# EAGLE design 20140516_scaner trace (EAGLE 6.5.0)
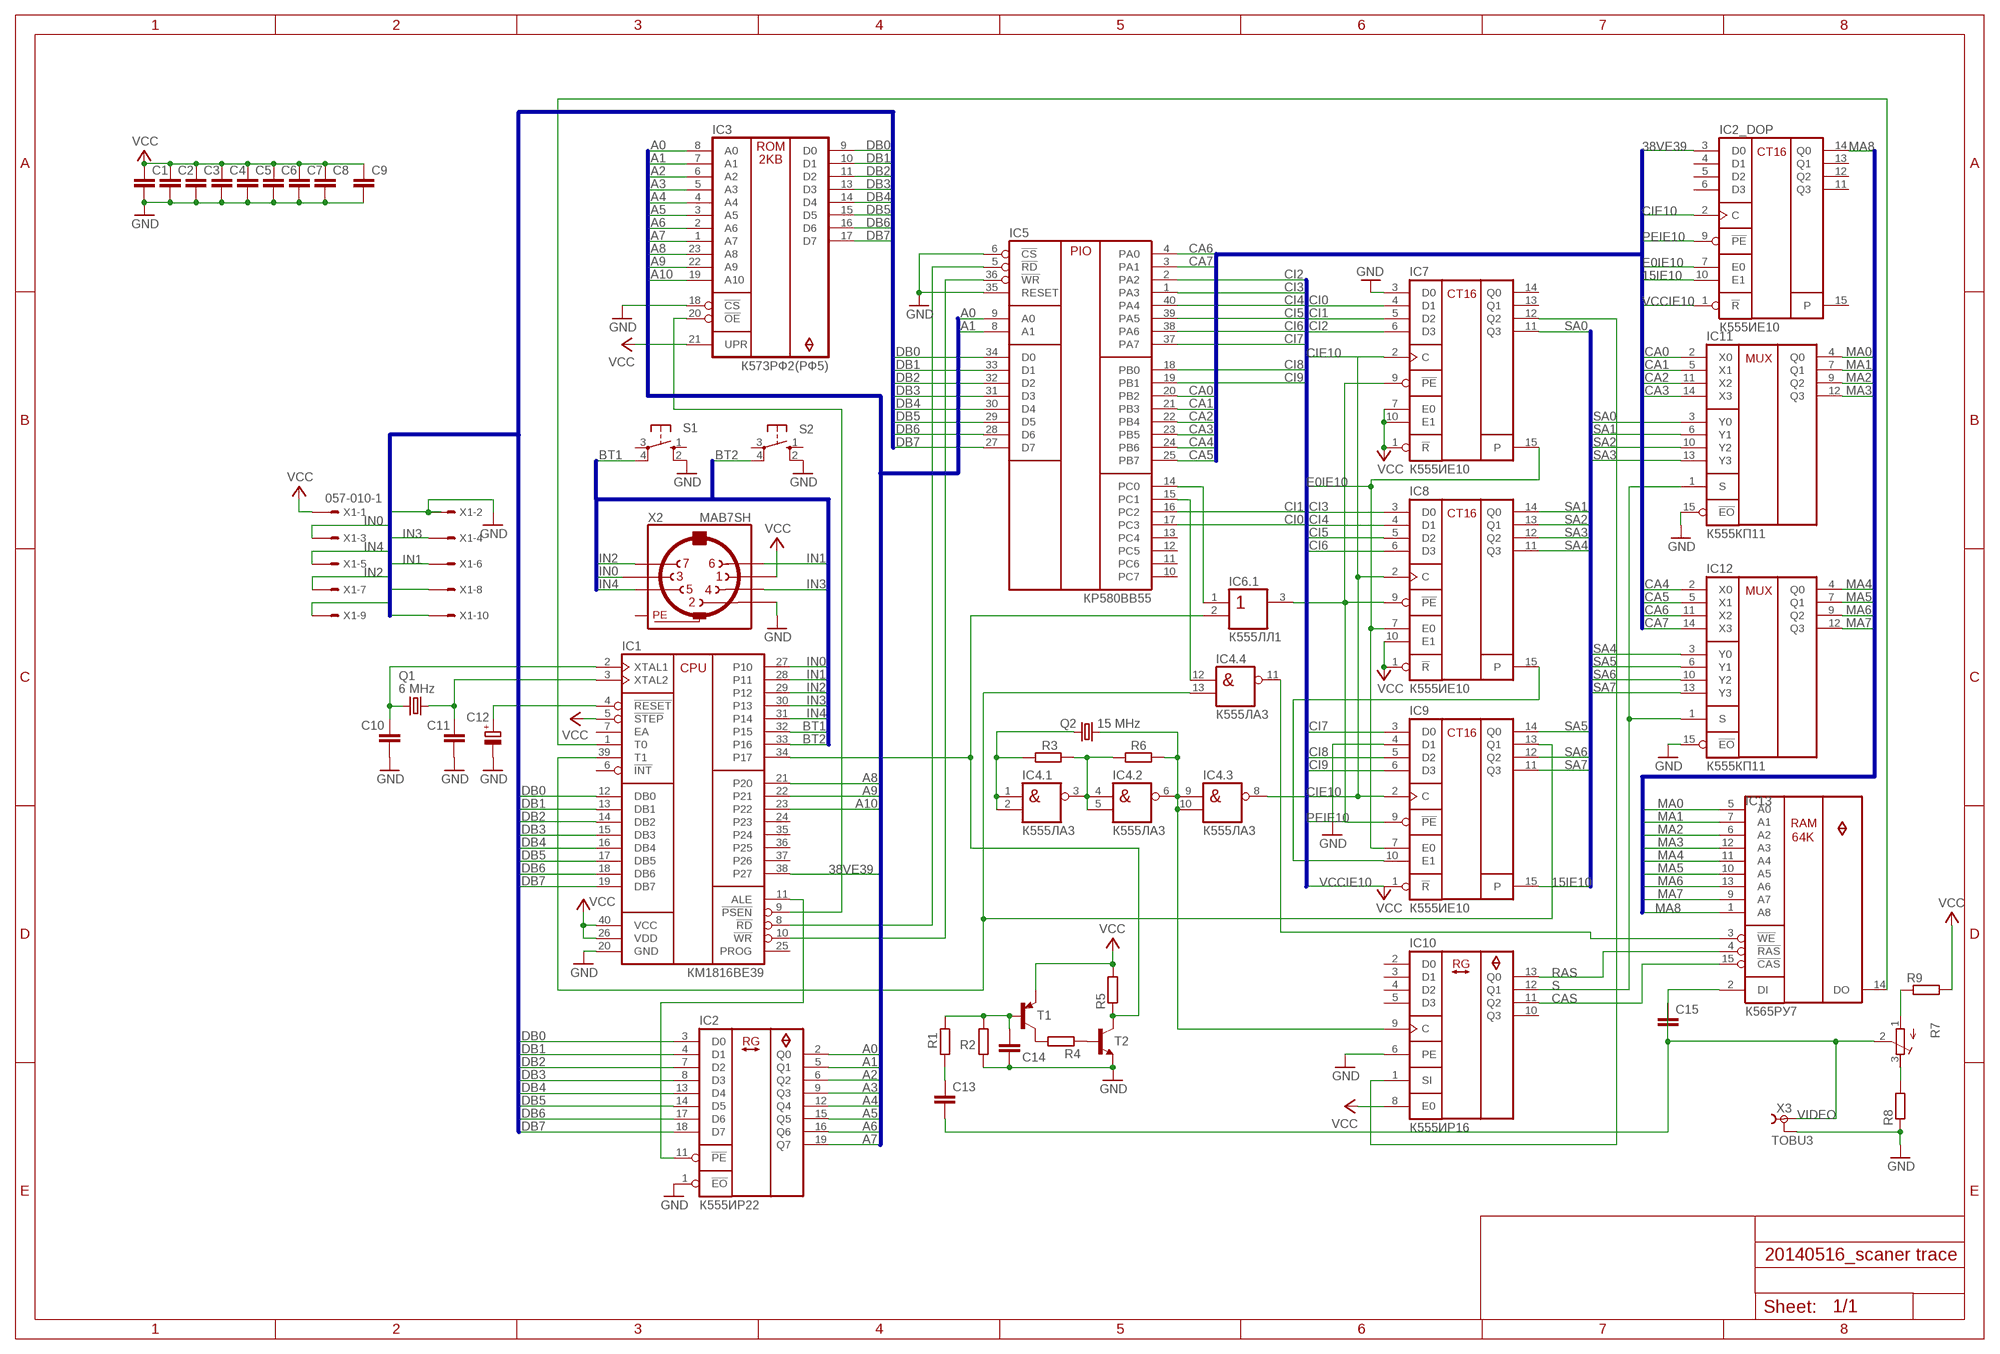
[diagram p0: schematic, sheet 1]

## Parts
C1  C-EU050-025X075  [C050-025X075]
C2  C-EU050-025X075  [C050-025X075]
C3  C-EU050-025X075  [C050-025X075]
C4  C-EU050-025X075  [C050-025X075]
C5  C-EU050-025X075  [C050-025X075]
C6  C-EU050-025X075  [C050-025X075]
C7  C-EU050-025X075  [C050-025X075]
C8  C-EU050-025X075  [C050-025X075]
C9  C-EU050-025X075  [C050-025X075]
C10  C-EU050-025X075  [C050-025X075]
C11  C-EU050-025X075  [C050-025X075]
C12  CPOL-EUE2,5-6E  [E2,5-6E]
C13  C-EU050-025X075  [C050-025X075]
C14  C-EU050-025X075  [C050-025X075]
C15  C-EU050-025X075  [C050-025X075]
IC1  КМ1816ВЕ39  [DIP40]
IC2  К555ИР22  [DIP20]
IC2_DOP  К555ИЕ10  [DIP16]
IC3  К573РФ2(РФ5)  К573РФ2  [DIP24]
IC4  К555ЛА3  [DIP14]
IC5  КР580ВВ55  [DIP40]
IC6  К555ЛЛ1  [DIP14]
IC7  К555ИЕ10  [DIP16]
IC8  К555ИЕ10  [DIP16]
IC9  К555ИЕ10  [DIP16]
IC10  К555ИР16  [DIP14]
IC11  К555КП11  [DIP16]
IC12  К555КП11  [DIP16]
IC13  К565РУ7  [DIP16]
Q1  6 MHz  CRYSTALZX_V  [HC49U_V_ZX]
Q2  15 MHz  CRYSTALZX_V  [HC49U_V_ZX]
R1  R-EU_  [0207/10_L17]
R2  R-EU_  [0207/10_L17]
R3  R-EU_  [0207/10_L17]
R4  R-EU_  [0207/10_L17]
R5  R-EU_  [0207/10_L17]
R6  R-EU_  [0207/10_L17]
R7  R-TRIMM3339P  [RTRIM3339P]
R8  R-EU_  [0207/10_L17]
R9  R-EU_  [0207/10_L17]
S1  40-XX  [B3F-40XX-LION17]
S2  40-XX  [B3F-40XX-LION17]
T1  -PNP-  [TO92-EBC-LION17]
T2  -NPN-  [KT315]
X1  057-010-1  [057-010-1]
X2  MAB7SH  [DIN7]
X3  TOBU3  [TOBU3]

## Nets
15IE10: IC2_DOP.10(E1) IC9.15(P)
38VE39: IC1.38(P27) IC2_DOP.3(D0)
A0: IC2.2(Q0) IC3.8(A0) IC5.9(A0)
A1: IC2.5(Q1) IC3.7(A1) IC5.8(A1)
A2: IC2.6(Q2) IC3.6(A2)
A3: IC2.9(Q3) IC3.5(A3)
A4: IC2.12(Q4) IC3.4(A4)
A5: IC2.15(Q5) IC3.3(A5)
A6: IC2.16(Q6) IC3.2(A6)
A7: IC2.19(Q7) IC3.1(A7)
A8: IC1.21(P20) IC3.23(A8)
A9: IC1.22(P21) IC3.22(A9)
A10: IC1.23(P22) IC3.19(A10)
BT1: IC1.32(P15) S1.4(P1)
BT2: IC1.33(P16) S2.4(P1)
CA0: IC5.20(PB2) IC11.2(X0)
CA1: IC5.21(PB3) IC11.5(X1)
CA2: IC5.22(PB4) IC11.11(X2)
CA3: IC5.23(PB5) IC11.14(X3)
CA4: IC5.24(PB6) IC12.2(X0)
CA5: IC5.25(PB7) IC12.5(X1)
CA6: IC5.4(PA0) IC12.11(X2)
CA7: IC5.3(PA1) IC12.14(X3)
CAS: IC10.11(Q2) IC13.15(!CAS)
CI0: IC5.17(PC3) IC7.4(D1)
CI1: IC5.16(PC2) IC7.5(D2)
CI2: IC5.2(PA2) IC7.6(D3)
CI3: IC5.1(PA3) IC8.3(D0)
CI4: IC5.40(PA4) IC8.4(D1)
CI5: IC5.39(PA5) IC8.5(D2)
CI6: IC5.38(PA6) IC8.6(D3)
CI7: IC5.37(PA7) IC9.3(D0)
CI8: IC5.18(PB0) IC9.5(D2)
CI9: IC5.19(PB1) IC9.6(D3)
CIE10: IC2_DOP.2(C) IC4.8(.3:OUT) IC7.2(C) IC8.2(C) IC9.2(C)
DB0: IC1.12(DB0) IC2.3(D0) IC3.9(D0) IC5.34(D0)
DB1: IC1.13(DB1) IC2.4(D1) IC3.10(D1) IC5.33(D1)
DB2: IC1.14(DB2) IC2.7(D2) IC3.11(D2) IC5.32(D2)
DB3: IC1.15(DB3) IC2.8(D3) IC3.13(D3) IC5.31(D3)
DB4: IC1.16(DB4) IC2.13(D4) IC3.14(D4) IC5.30(D4)
DB5: IC1.17(DB5) IC2.14(D5) IC3.15(D5) IC5.29(D5)
DB6: IC1.18(DB6) IC2.17(D6) IC3.16(D6) IC5.28(D6)
DB7: IC1.19(DB7) IC2.18(D7) IC3.17(D7) IC5.27(D7)
E0IE10: IC2_DOP.7(E0) IC7.15(P) IC8.7(E0) IC9.7(E0)
GND [GND]: C1.2 C2.2 C3.2 C4.2 C5.2 C6.2 C7.2 C8.2 C9.2 C10.2 C11.2 C12.- C14.2 IC1.20(GND) IC2.1(!EO) IC3.18(!CS) IC5.6(!CS) IC5.35(RESET) IC7.3(D0) IC9.4(D1) IC10.6(PE) IC11.15(!EO) IC12.15(!EO) R2.1 R8.1 S1.2(S1) S2.2(S1) T2.E X1.2 X2.2 X3.2 X3.2@1 X3.2@2
IN0: IC1.27(P10) X1.3 X2.3
IN1: IC1.28(P11) X1.6 X2.6
IN2: IC1.29(P12) X1.7 X2.7
IN3: IC1.30(P13) X1.4 X2.4
IN4: IC1.31(P14) X1.5 X2.5
MA0: IC11.4(Q0) IC13.5(A0)
MA1: IC11.7(Q1) IC13.7(A1)
MA2: IC11.9(Q2) IC13.6(A2)
MA3: IC11.12(Q3) IC13.12(A3)
MA4: IC12.4(Q0) IC13.11(A4)
MA5: IC12.7(Q1) IC13.10(A5)
MA6: IC12.9(Q2) IC13.13(A6)
MA7: IC12.12(Q3) IC13.9(A7)
MA8: IC2_DOP.14(Q0) IC13.1(A8)
N$1: IC8.15(P) IC9.10(E1)
N$4: C13.2 C15.2
N$6: X1.9
N$11: X1.8
N$12: X1.10
N$14: IC7.12(Q2) IC10.1(SI)
N$15: IC4.1(.1:IN1) IC4.2(.1:IN2) Q2.1 R3.1
N$16: IC4.3(.1:OUT) IC4.4(.2:IN1) IC4.5(.2:IN2) R3.2 R6.1
N$17: IC4.6(.2:OUT) IC4.9(.3:IN1) IC4.10(.3:IN2) IC10.9(C) Q2.2 R6.2
N$38: IC5.14(PC0) IC6.1(.1:IN1)
N$39: IC4.12(.4:IN1) IC5.15(PC1)
N$66: IC1.1(T0) IC13.14(DO)
N$67: C13.1 R1.2
N$69: R7.3(A) R8.2
N$70: R7.1(E) R9.1
N$71: C14.1 R1.1 R2.2 T1.B
N$72: C10.1 IC1.2(XTAL1) Q1.1
N$73: IC1.39(T1) IC4.13(.4:IN2) IC9.13(Q1)
N$74: C11.1 IC1.3(XTAL2) Q1.2
N$75: C12.+ IC1.4(!RESET)
N$76: IC1.8(!RD) IC5.5(!RD)
N$77: IC1.9(!PSEN) IC3.20(!OE)
N$78: IC1.10(!WR) IC5.36(!WR)
N$79: IC1.11(ALE) IC2.11(!PE)
N$85: IC1.34(P17) IC6.2(.1:IN2) R5.1 T2.C
N$86: R4.1 T2.B
N$87: R4.2 T1.C
PEIE10: IC2_DOP.9(!PE) IC6.3(.1:OUT) IC7.9(!PE) IC8.9(!PE) IC9.9(!PE)
RAS: IC10.13(Q0) IC13.4(!RAS)
S: IC10.12(Q1) IC11.1(S) IC12.1(S)
SA0: IC7.11(Q3) IC11.3(Y0)
SA1: IC8.14(Q0) IC11.6(Y1)
SA2: IC8.13(Q1) IC11.10(Y2)
SA3: IC8.12(Q2) IC11.13(Y3)
SA4: IC8.11(Q3) IC12.3(Y0)
SA5: IC9.14(Q0) IC12.6(Y1)
SA6: IC9.12(Q2) IC12.10(Y2)
SA7: IC9.11(Q3) IC12.13(Y3)
VCC [+5V]: C1.1 C2.1 C3.1 C4.1 C5.1 C6.1 C7.1 C8.1 C9.1 IC1.5(!STEP) IC1.26(VDD) IC1.40(VCC) IC3.21(UPR) IC7.1(!R) IC7.7(E0) IC7.10(E1) IC8.1(!R) IC8.10(E1) IC10.8(E0) R5.2 R9.2 T1.E X1.1 X2.1
VCCIE10: IC2_DOP.1(!R) IC9.1(!R) ; supply symbol labelled VCC
VIDEO: C15.1 IC13.2(DI) R7.2(S) X3.1
WE: IC4.11(.4:OUT) IC13.3(!WE)
Unconnected: IC1.6(!INT) IC1.7(EA) IC1.24(P23) IC1.25(PROG) IC1.35(P24) IC1.36(P25) IC1.37(P26) IC2_DOP.4(D1) IC2_DOP.5(D2) IC2_DOP.6(D3) IC2_DOP.11(Q3) IC2_DOP.12(Q2) IC2_DOP.13(Q1) IC2_DOP.15(P) IC5.10(PC7) IC5.11(PC6) IC5.12(PC5) IC5.13(PC4) IC6.4(.2:IN1) IC6.5(.2:IN2) IC6.6(.2:OUT) IC6.8(.3:OUT) IC6.9(.3:IN1) IC6.10(.3:IN2) IC6.11(.4:OUT) IC6.12(.4:IN1) IC6.13(.4:IN2) IC7.13(Q1) IC7.14(Q0) IC10.2(D0) IC10.3(D1) IC10.4(D2) IC10.5(D3) IC10.10(Q3) S1.1(S) S1.3(P) S2.1(S) S2.3(P) X2.PE X2.PE1(PE) X2.PE@1(PE) X2.PE@(PE)

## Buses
DB[0..7]
MA[0..7]
CA[0..7]
SA[0..7]
CI[0..9]
A[0..10]
IN[0..4],BT[1..2]

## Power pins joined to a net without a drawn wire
GND: IC2.10(GND) IC2_DOP.8(GND) IC3.12(GND) IC4.7(GND) IC5.7(GND) IC6.7(GND) IC7.8(GND) IC8.8(GND) IC9.8(GND) IC10.7(GND) IC11.8(GND) IC12.8(GND)
VCC: IC2.20(VCC) IC2_DOP.16(VCC) IC3.24(VCC) IC4.14(VCC) IC5.26(VCC) IC6.14(VCC) IC7.16(VCC) IC8.16(VCC) IC9.16(VCC) IC10.14(VCC) IC11.16(VCC) IC12.16(VCC)

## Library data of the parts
C1-C11 C13-C15 = rcl:C-EU: CAPACITOR, European symbol
C12 = rcl:CPOL-EU: POLARIZED CAPACITOR, European symbol
IC1 = lion17:КМ1816ВЕ39
IC2 = lion17:К555ИР22
IC2_DOP = _lion17:К555ИЕ10
IC3 = lion17:К573РФ2
IC4 = lion17:К555ЛА3
IC5 = lion17:КР580ВВ55
IC6 = lion17:К555ЛЛ1
IC7-IC9 = lion17:К555ИЕ10
IC10 = lion17:К555ИР16
IC11 IC12 = lion17:К555КП11
IC13 = _lion17:К565РУ7
Q1 Q2 = crystal:CRYSTAL: CRYSTAL
R1-R6 R8 R9 = rcl:R-EU_: RESISTOR, European symbol
R7 = resistor:R-TRIMM: Trimm resistor
S1 S2 = switch-omron:40-XX: OMRON SWITCH
T1 = transistor-neu-to92:*-PNP-: PNP Transistror
T2 = transistor-neu-to92:*-NPN-: NPN Transistror
X1 = con-panduit:057-010-: CONNECTOR 10-pin series 057 contact pc board low profile headers; OC_FARNELL: unknown; OC_NEWARK: unknown
X2 = con-hirschmann:MAB7SH: Female CONNECTOR 7 pins with shield, horizontal (DIN 45329)
X3 = con-hirschmann:TOBU3: Female Cinch CONNECTOR ( RCA Jack ); MF: FARNELL; MPN: TOBU 3; OC_FARNELL: 592791; OC_NEWARK: 06WX5914

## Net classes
0 default: clearance 0.205 mm
1 GND: width 0.203 mm, clearance 0.205 mm to class 0, clearance 0.205 mm
2 +5V: width 0.203 mm, clearance 0.205 mm to class 0, clearance 0.205 mm to class 1, clearance 0.205 mm

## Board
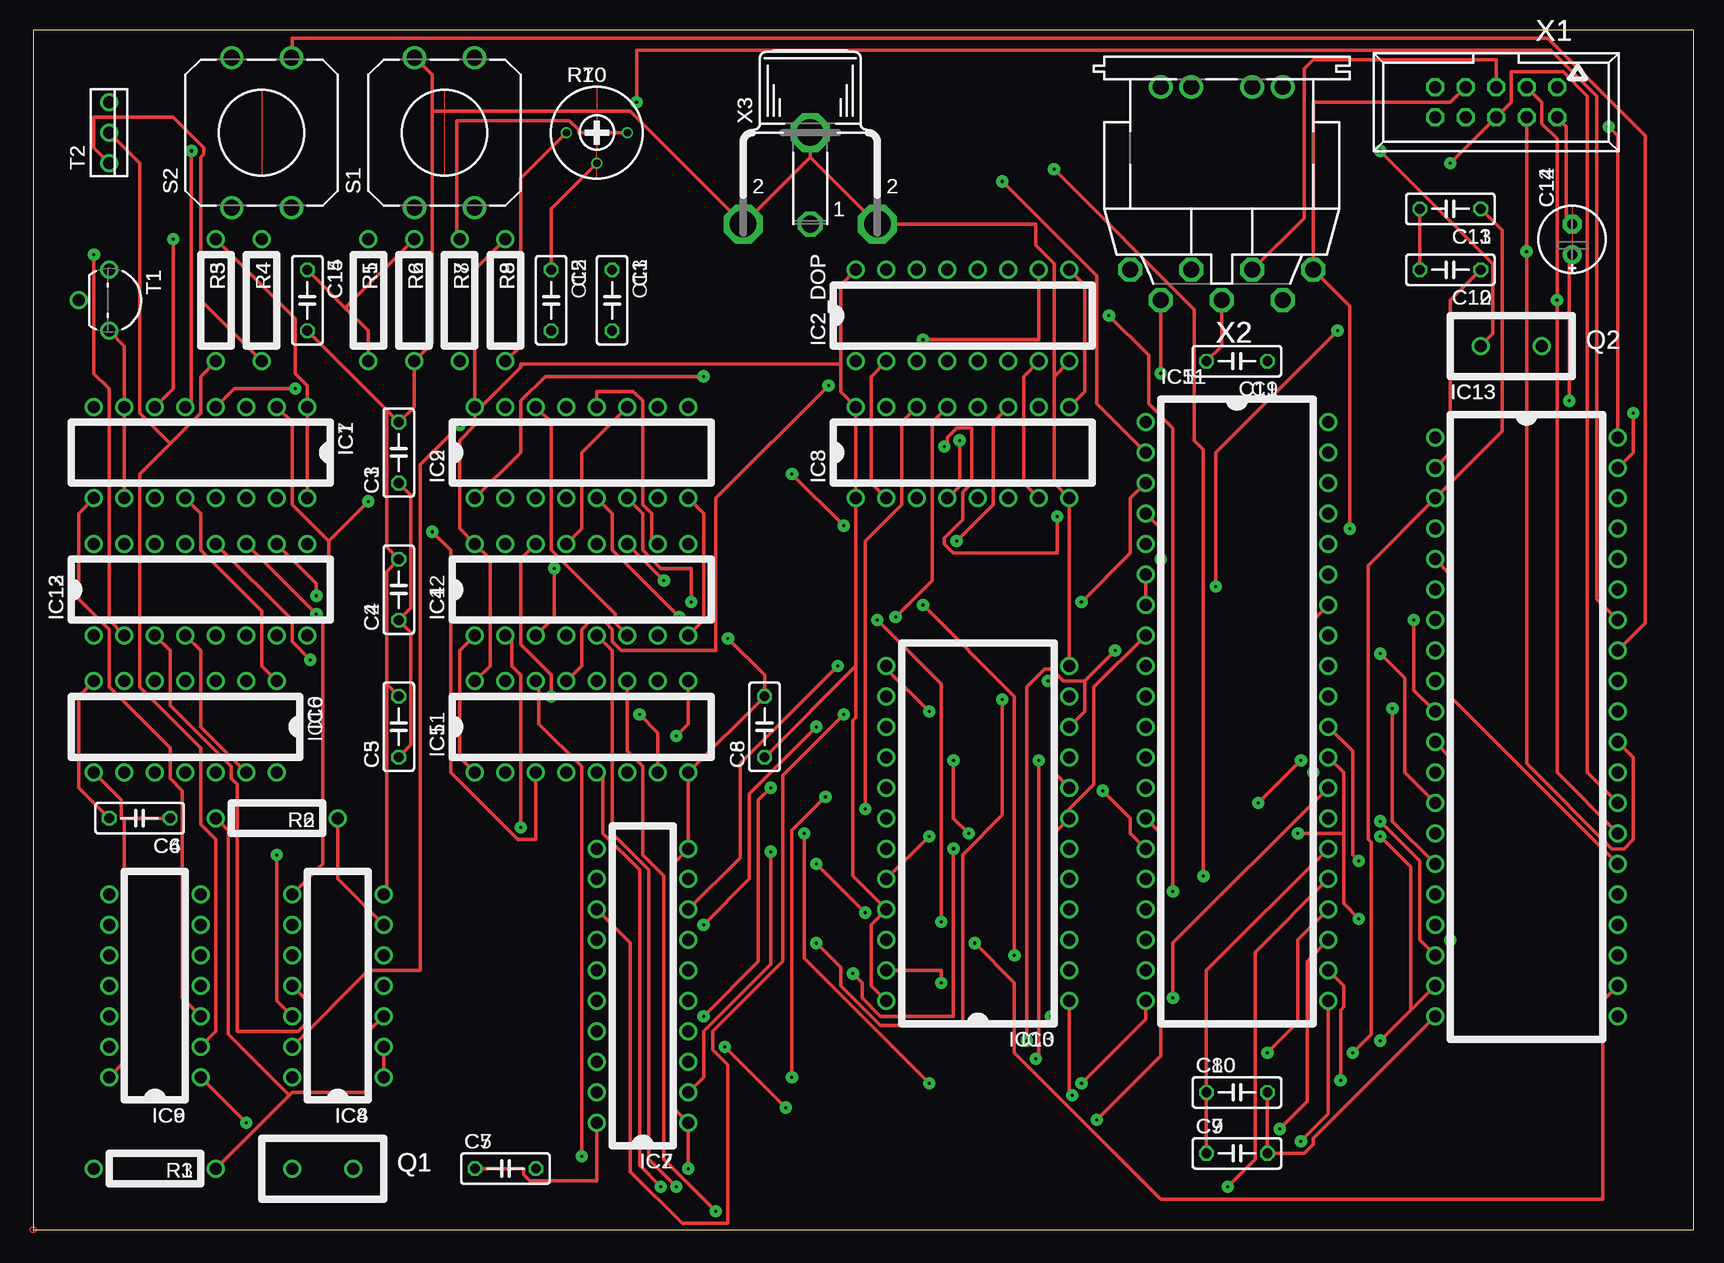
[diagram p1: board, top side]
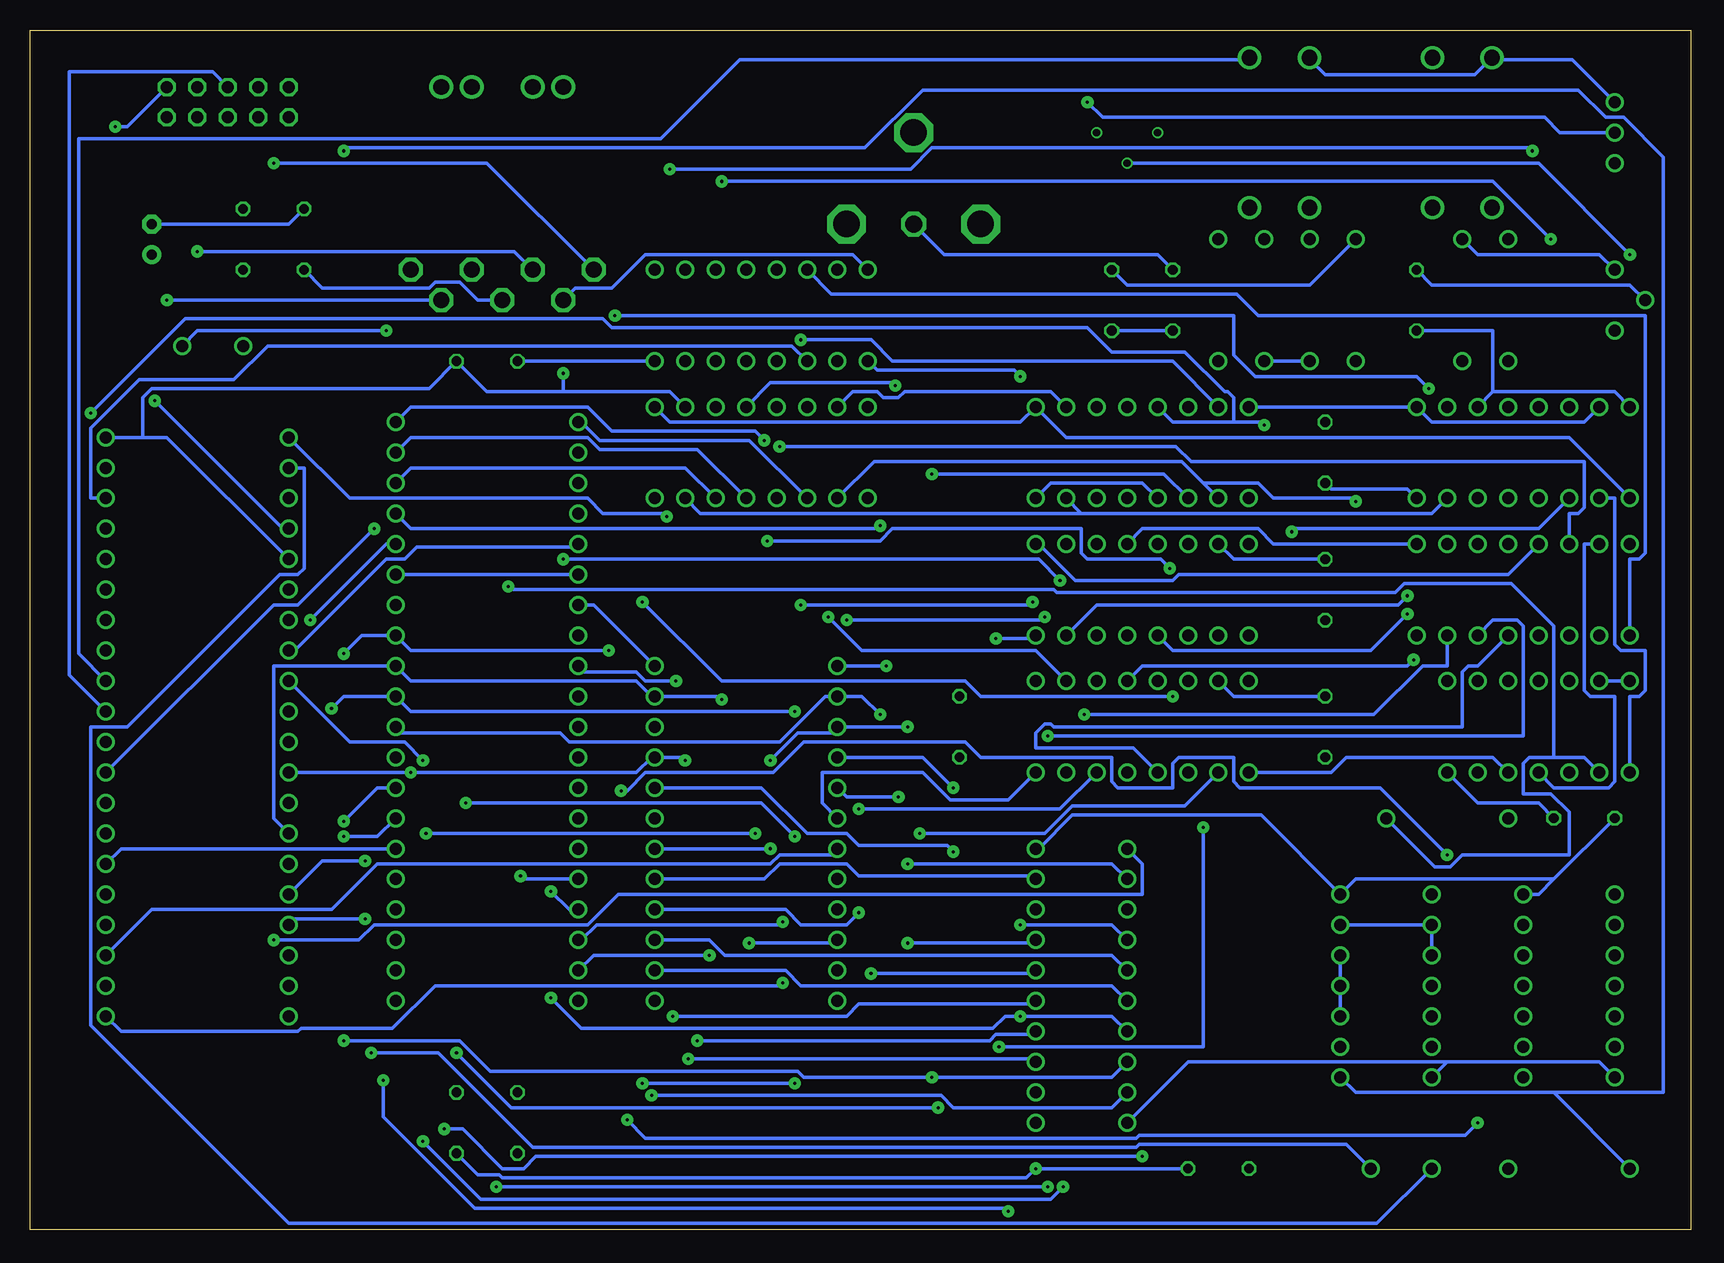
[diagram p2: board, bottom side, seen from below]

Size 138.41 x 100 mm. Coordinates in mm from the lower left corner, seen from the top.
Outline: 0,0 138.41,0 138.41,100 0,100 0,0
Copper layers (1*16): Top 0.035mm / dielectric 1.5mm / Bottom 0.035mm
Design rules "20140516_scaner trace": minimum track width 12mil, minimum drill 10mil, track to track 0.205mm, track to pad 0.205mm, pad to pad 0.205mm, via to via 0.205mm, smd to smd 8mil, copper to edge 10mil, drill to drill 20mil, minimum pad ring 5mil, minimum via ring 15mil, stop-mask expansion 4mil, vias tented up to drill 0mil, thermal gap 10mil

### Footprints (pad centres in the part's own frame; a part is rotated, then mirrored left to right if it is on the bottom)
C050-025X075 = drill 0.813 octagon: 1 -2.54,0; 2 2.54,0
E2,5-6E = drill 0.813 pad 1.575: + -1.27,0 | drill 0.813 pad 1.575 octagon: - 1.27,0
DIP40 = drill 1 pad 1.422: 1 -7.62,2.54; 2 -7.62,0; 3 -7.62,-2.54; 4 -7.62,-5.08; 5 -7.62,-7.62; 6 -7.62,-10.16; 7 -7.62,-12.7; 8 -7.62,-15.24; 9 -7.62,-17.78; 10 -7.62,-20.32; 11 -7.62,-22.86; 12 -7.62,-25.4; 13 -7.62,-27.94; 14 -7.62,-30.48; 15 -7.62,-33.02; 16 -7.62,-35.56; 17 -7.62,-38.1; 18 -7.62,-40.64; 19 -7.62,-43.18; 20 -7.62,-45.72; 21 7.62,-45.72; 22 7.62,-43.18; 24 7.62,-38.1; 25 7.62,-35.56; 26 7.62,-33.02; 27 7.62,-30.48; 28 7.62,-27.94; 29 7.62,-25.4; 30 7.62,-22.86; 31 7.62,-20.32; 32 7.62,-17.78; 33 7.62,-15.24; 34 7.62,-12.7; 35 7.62,-10.16; 36 7.62,-7.62; 37 7.62,-5.08; 38 7.62,-2.54; 39 7.62,0; 40 7.62,2.54 | drill 1: 23 7.62,-40.64
DIP20 = drill 1 pad 1.422: 1 -3.81,1.27; 2 -3.81,-1.27; 3 -3.81,-3.81; 4 -3.81,-6.35; 5 -3.81,-8.89; 6 -3.81,-11.43; 7 -3.81,-13.97; 8 -3.81,-16.51; 9 -3.81,-19.05; 10 -3.81,-21.59; 11 3.81,-21.59; 12 3.81,-19.05; 13 3.81,-16.51; 14 3.81,-13.97; 15 3.81,-11.43; 16 3.81,-8.89; 17 3.81,-6.35; 18 3.81,-3.81; 19 3.81,-1.27; 20 3.81,1.27
DIP16 = drill 1 pad 1.422: 1 -3.81,1.27; 2 -3.81,-1.27; 3 -3.81,-3.81; 4 -3.81,-6.35; 5 -3.81,-8.89; 6 -3.81,-11.43; 7 -3.81,-13.97; 8 -3.81,-16.51; 9 3.81,-16.51; 10 3.81,-13.97; 11 3.81,-11.43; 12 3.81,-8.89; 13 3.81,-6.35; 14 3.81,-3.81; 15 3.81,-1.27; 16 3.81,1.27
DIP24 = drill 1 pad 1.422: 1 -7.62,1.27; 2 -7.62,-1.27; 3 -7.62,-3.81; 4 -7.62,-6.35; 5 -7.62,-8.89; 6 -7.62,-11.43; 7 -7.62,-13.97; 8 -7.62,-16.51; 9 -7.62,-19.05; 10 -7.62,-21.59; 11 -7.62,-24.13; 12 -7.62,-26.67; 13 7.62,-26.67; 14 7.62,-24.13; 15 7.62,-21.59; 16 7.62,-19.05; 17 7.62,-16.51; 18 7.62,-13.97; 19 7.62,-11.43; 20 7.62,-8.89; 21 7.62,-6.35; 22 7.62,-3.81; 23 7.62,-1.27; 24 7.62,1.27
DIP14 = drill 1 pad 1.422: 1 -3.81,1.27; 2 -3.81,-1.27; 3 -3.81,-3.81; 4 -3.81,-6.35; 5 -3.81,-8.89; 6 -3.81,-11.43; 7 -3.81,-13.97; 8 3.81,-13.97; 9 3.81,-11.43; 10 3.81,-8.89; 11 3.81,-6.35; 12 3.81,-3.81; 13 3.81,-1.27; 14 3.81,1.27
HC49U_V_ZX = drill 1 pad 1.422: 1 -2.54,0; 2 2.54,0
0207/10_L17 = drill 1 pad 1.422: 1 -5.08,0; 2 5.08,0
RTRIM3339P = drill 0.61: 1 -2.54,0; 2 0,-2.54; 3 2.54,0
B3F-40XX-LION17 = drill 1.3: 1 -6.248,2.489; 2 6.248,2.489; 3 -6.248,-2.489; 4 6.248,-2.489
TO92-EBC-LION17 = drill 1 pad 1.422: B 0,-2.54; C -2.54,0; E 2.54,0
KT315 = drill 1 pad 1.422: B -2.54,0; C 0,0; E 2.54,0
057-010-1 = drill 1 octagon: 1 -5.08,-1.27; 2 -5.08,1.27; 3 -2.54,-1.27; 4 -2.54,1.27; 5 0,-1.27; 6 0,1.27; 7 2.54,-1.27; 8 2.54,1.27; 9 5.08,-1.27; 10 5.08,1.27
DIN7 = drill 1.321 octagon: 1 5.08,12.7; 2 0,12.7; 3 -5.08,12.7; 4 2.54,10.16; 5 -2.54,10.16; 6 7.62,10.16; 7 -7.62,10.16 | drill 1.321: PE -2.54,-5.08; PE1 -5.08,-5.08; PE@ 2.54,-5.08; PE@1 5.08,-5.08
TOBU3 = drill 1.397 octagon: 1 0,-2.54 | drill 2.21 octagon: 2 5.588,-2.54; 2@1 -5.588,-2.54; 2@2 0,5.08

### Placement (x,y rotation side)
C1  30.48,64.77 90 top
C2  30.48,53.34 90 top
C3  30.48,41.91 90 top
C4  8.89,34.29 180 top
C5  39.37,5.08 0 top
C6  60.96,41.91 90 top
C7  100.33,6.35 0 top
C8  100.33,11.43 0 top
C9  100.33,72.39 180 top
C10  118.11,80.01 180 top
C11  118.11,85.09 180 top
C12  128.27,82.55 90 top
C13  48.26,77.47 270 top
C14  22.86,77.47 270 top
C15  43.18,77.47 270 top
DRILEGEND  [DRILEGEND]  not placed on the board
IC1  124.46,63.5 0 top
IC2  50.8,10.16 180 top
IC2_DOP  69.85,76.2 90 top
IC3  78.74,20.32 180 top
IC4  25.4,13.97 180 top
IC5  100.33,64.77 0 top
IC6  10.16,13.97 180 top
IC7  21.59,64.77 270 top
IC8  69.85,64.77 90 top
IC9  38.1,64.77 90 top
IC10  19.05,41.91 270 top
IC11  38.1,41.91 90 top
IC12  38.1,53.34 90 top
IC13  6.35,53.34 90 top
Q1  24.13,5.08 0 top
Q2  123.19,73.66 0 top
R1  27.94,77.47 90 top
R2  31.75,77.47 90 top
R3  10.16,5.08 0 top
R4  19.05,77.47 90 top
R5  15.24,77.47 90 top
R6  20.32,34.29 0 top
R7  46.99,91.44 0 top
R8  35.56,77.47 90 top
R9  39.37,77.47 90 top
S1  34.29,91.44 90 top
S2  19.05,91.44 90 top
T1  6.35,77.47 270 top
T2  6.35,91.44 90 top
X1  121.92,93.98 180 top
X2  99.06,90.17 180 top
X3  64.77,86.36 0 top

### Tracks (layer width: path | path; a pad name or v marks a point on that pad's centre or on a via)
15IE10  (via drill 0.25)
  Top 0.305: v74.17,74.17 83.82,74.17 IC2_DOP.10
  Bottom 0.305: IC9.15 43.18,72.39 66.55,72.39 68.33,74.17 v74.17,74.17
38VE39
  Bottom 0.305: IC2_DOP.3 74.93,73.66 118.62,73.66 121.41,70.87 129.29,70.87 133.35,66.8 133.35,60.96 IC1.38
A0  (via drill 0.25)
  Top 0.305: IC2.2 55.88,12.7 55.88,16.51 61.47,22.1 v61.47,31.5 | v84.58,45.72 85.09,45.21 85.09,38.1 IC3.8
  Bottom 0.305: v61.47,31.5 61.98,32 69.34,32 70.36,33.02 73.66,33.02 77.47,36.83 IC3.8 | IC5.9 92.2,46.48 87.88,46.48 87.12,45.72 v84.58,45.72
A1  (via drill 0.25)
  Top 0.305: v84.84,17.78 85.09,18.03 85.09,33.02 IC3.7 86.36,35.05 88.39,37.08 88.39,45.21 IC5.8
  Bottom 0.305: IC2.5 54.86,18.8 69.34,18.8 70.36,17.78 v84.84,17.78
A2  (via drill 0.25)
  Top 0.305: v68.33,21.34 69.09,20.57 69.09,19.3 70.61,17.78 76.71,17.78 v76.71,31.75
  Bottom 0.305: IC2.6 54.86,21.34 v68.33,21.34 | IC3.6 v76.71,31.75
A3
  Bottom 0.305: IC2.9 54.86,29.46 69.34,29.46 70.36,30.48 75.95,30.48 77.22,29.21 IC3.5
A4  (via drill 0.25)
  Top 0.305: v69.34,26.42 v65.28,30.48
  Bottom 0.305: IC2.12 48.26,30.48 v65.28,30.48 | v69.34,26.42 70.36,25.4 74.17,25.4 75.44,26.67 IC3.4
A5
  Bottom 0.305: IC2.15 48.26,22.86 80.52,22.86 81.79,24.13 IC3.3
A6
  Bottom 0.305: IC2.16 48.26,20.32 74.17,20.32 75.44,21.59 IC3.2
A7  (via drill 0.25)
  Top 0.305: v86.61,11.18 86.36,11.43 IC3.1
  Bottom 0.305: IC2.19 48.26,10.16 61.47,10.16 62.48,11.18 v86.61,11.18
A8  (via drill 0.25)
  Top 0.305: IC3.23 75.69,21.59 v75.69,20.57
  Bottom 0.305: v75.69,20.57 75.95,20.32 104.65,20.32 108.2,16.76 115.82,16.76 116.08,16.51 130.81,16.51 IC1.21
A9  (via drill 0.25)
  Top 0.305: v78.49,23.88 81.79,20.57 81.79,14.73 93.98,2.54 130.81,2.54 130.81,19.05 IC1.22
  Bottom 0.305: IC3.22 71.37,23.88 v78.49,23.88
A10
  Bottom 0.305: IC3.19 71.63,31.24 75.95,31.24 76.71,30.48 109.47,30.48 113.28,26.67 128.27,26.67 IC1.23
BT1
  Bottom 0.305: IC1.32 134.37,48.01 134.37,90.93 85.85,90.93 79.25,97.54 36.83,97.54 S1.4
BT2
  Top 0.305: IC1.33 134.37,50.55 134.37,91.19 126.24,99.31 21.59,99.31 21.59,97.79 S2.4
CA0  (via drill 0.25)
  Top 0.305: v64.26,33.02 64.26,22.61 v74.68,12.19 | v87.38,12.19 92.71,17.53 IC5.20
  Bottom 0.305: IC11.2 42.16,35.31 51.56,35.31 53.85,33.02 v64.26,33.02 | v87.38,12.19 v74.68,12.19
CA1  (via drill 0.25)
  Top 0.305: IC11.5 47.5,37.59 47.5,33.02 50.55,29.97 50.55,5.33 v52.32,3.56 | v105.66,7.37 107.95,9.65 IC5.21
  Bottom 0.305: v52.32,3.56 53.34,2.54 100.84,2.54 v105.66,7.37
CA2  (via drill 0.25)
  Top 0.305: IC11.11 49.53,39.88 50.8,38.61 50.8,31.24 52.58,29.46 52.58,5.84 v56.9,1.52 | v108.97,12.45 108.97,18.29 109.22,18.54 109.22,20.32 IC5.22
  Bottom 0.305: v56.9,1.52 57.15,1.78 101.35,1.78 108.97,9.4 v108.97,12.45
CA3  (via drill 0.25)
  Top 0.305: IC11.14 42.16,45.47 42.16,42.16 45.72,38.61 v45.72,6.1 | v103.89,8.38 106.17,10.67 106.17,22.35 IC5.23
  Bottom 0.305: v45.72,6.1 96.27,6.1 97.28,5.08 99.06,5.08 102.36,8.38 v103.89,8.38
CA4  (via drill 0.25)
  Top 0.305: IC12.2 39.88,49.02 39.88,46.99 40.64,46.23 v40.64,33.53 | v62.74,10.16 v57.66,15.24 | v102.87,14.73 105.41,17.27 105.41,24.13 IC5.24
  Bottom 0.305: v40.64,33.53 40.64,15.24 v57.66,15.24 | v62.74,10.16 98.3,10.16 v102.87,14.73
CA5  (via drill 0.25)
  Top 0.305: IC12.5 48.26,48.26 48.26,33.02 51.31,29.97 51.31,5.84 v53.59,3.56 | v99.57,3.56 101.85,5.84 101.85,23.11 IC5.25
  Bottom 0.305: v99.57,3.56 v53.59,3.56
CA6  (via drill 0.25)
  Top 0.305: v52.58,54.1 IC12.11 | v93.98,55.88 93.98,58.42 IC5.4
  Bottom 0.305: v52.58,54.1 54.36,55.88 v93.98,55.88
CA7  (via drill 0.25)
  Top 0.305: IC12.14 40.64,55.88 40.64,48.77 43.18,46.23 v43.18,44.45 | v87.38,52.32 91.44,56.39 91.44,60.96 IC5.3
  Bottom 0.305: v43.18,44.45 59.18,44.45 60.45,45.72 80.77,45.72 v87.38,52.32
CAS
  Bottom 0.305: IC10.11 11.43,36.83 6.86,36.83 6.35,37.34 6.35,44.45 8.38,44.45 8.89,44.96 8.89,57.15 IC13.15
CI0  (via drill 0.25)
  Top 0.305: IC7.4 16.76,70.1 v21.84,70.1 | v89.66,76.2 92.96,72.9 92.96,68.83 95,66.8 v95,28.19
  Bottom 0.305: v21.84,70.1 22.86,71.12 36.32,71.12 38.1,72.9 38.1,76.2 v89.66,76.2 | v95,28.19 93.47,26.67 IC5.17
CI1  (via drill 0.25)
  Top 0.305: IC7.5 13.21,69.09 v13.21,89.92 | v85.09,88.39 96.77,76.71 96.77,65.79 97.54,65.02 v97.54,29.46
  Bottom 0.305: v13.21,89.92 13.46,90.17 63.25,90.17 65.02,88.39 v85.09,88.39 | v97.54,29.46 97.28,29.21 IC5.16
CI2  (via drill 0.25)
  Top 0.305: IC7.6 11.68,70.1 v11.68,82.55 | v80.77,87.38 88.65,79.5 88.65,68.83 IC5.2
  Bottom 0.305: v11.68,82.55 16.51,87.38 v80.77,87.38
CI3
  Bottom 0.305: IC8.3 78.49,65.79 90.93,65.79 92.46,67.31 IC5.1
CI4  (via drill 0.25)
  Top 0.305: IC8.4 77.22,61.98 v77.22,65.79
  Bottom 0.305: v77.22,65.79 77.98,66.55 89.92,66.55 91.95,68.58 106.68,68.58 IC5.40
CI5
  Bottom 0.305: IC8.5 82.8,65.02 90.93,65.02 91.95,66.04 106.68,66.04 IC5.39
CI6
  Bottom 0.305: IC8.6 83.82,63.5 106.68,63.5 IC5.38
CI7  (via drill 0.25)
  Top 0.305: v67.56,58.67 v63.25,62.99
  Bottom 0.305: IC9.3 43.94,62.99 v63.25,62.99 | v67.56,58.67 67.82,58.42 106.68,58.42 IC5.37
CI8  (via drill 0.25)
  Top 0.305: IC9.5 48.26,59.69 48.26,56.64 v53.85,51.05 | v70.36,50.8 75.69,45.47 v75.69,25.65
  Bottom 0.305: v53.85,51.05 54.1,50.8 v70.36,50.8 | v75.69,25.65 75.95,25.4 91.19,25.4 92.46,24.13 IC5.18
CI9  (via drill 0.25)
  Top 0.305: IC9.6 50.8,59.69 50.8,56.64 52.32,55.12 54.86,55.12 v54.86,52.32 | v74.17,52.07 81.79,44.45 v81.79,22.86
  Bottom 0.305: v54.86,52.32 55.12,52.07 v74.17,52.07 | v81.79,22.86 91.44,22.86 IC5.19
CIE10  (via drill 0.25)
  Top 0.305: IC4.8 24.13,30.48 24.13,50.55 24.64,51.05 24.64,57.4 | 24.64,57.4 21.59,60.45 21.59,67.31 IC7.2 | IC2_DOP.2 69.85,71.12 69.85,62.23 IC8.2 | v27.94,60.71 24.64,57.4
  Bottom 0.305: 40.64,62.23 42.42,64.01 68.07,64.01 IC8.2 | 40.64,62.23 IC9.2 | v27.94,60.71 28.19,60.96 34.8,60.96 36.07,62.23 40.64,62.23
DB0  (via drill 0.25)
  Top 0.305: v83.57,14.22 83.82,14.48 v83.82,39.12 | IC5.34 106.68,50.8 v106.68,38.1
  Bottom 0.305: IC2.3 54.86,14.22 v83.57,14.22 | v83.82,39.12 84.07,39.37 IC3.9 86.61,39.37 87.88,38.1 v106.68,38.1 IC1.12
DB1  (via drill 0.25)
  Top 0.305: IC1.13 114.3,38.1 114.3,45.97 v112.27,48.01 | v82.8,15.75 82.8,45.21 84.33,46.74 85.09,46.74 85.09,46.48 85.85,45.72 87.63,45.72 | 87.63,45.72 87.63,43.18 IC3.10 | 87.63,45.72 v90.17,48.26
  Bottom 0.305: v112.27,48.01 110.74,49.53 IC5.33 106.68,48.26 v90.17,48.26 | IC2.4 54.86,16.26 57.91,16.26 58.42,15.75 v82.8,15.75
DB2  (via drill 0.25)
  Top 0.305: v65.28,23.88 67.31,21.84 67.31,20.32 70.61,17.02 77.47,17.02 77.47,31.24 80.77,34.54 v80.77,44.2
  Bottom 0.305: IC2.7 54.86,23.88 v65.28,23.88 | v80.77,44.2 81.03,44.45 IC3.11 86.61,44.45 87.88,45.72 106.68,45.72 IC5.32 118.11,46.99 118.11,34.29 IC1.14
DB3  (via drill 0.25)
  Top 0.305: IC1.15 113.28,34.04 v113.28,43.43 | IC2.8 58.93,30.99 58.93,38.86 v67.06,46.99 | v74.68,43.18 71.12,46.74 IC3.13
  Bottom 0.305: v113.28,43.43 112.27,44.45 IC5.31 106.68,43.18 v74.68,43.18 | IC3.13 v67.06,46.99
DB4  (via drill 0.25)
  Top 0.305: IC2.13 49.78,23.88 49.78,4.83 54.1,0.51 57.91,0.51 57.91,13.72 56.64,14.99 56.64,16.51 62.48,22.35 62.48,37.85 v67.56,42.93 | v110.49,30.73 109.98,31.24 109.98,39.88 IC5.30
  Bottom 0.305: v67.56,42.93 69.09,44.45 IC3.14 72.14,44.45 75.95,40.64 93.47,40.64 94.23,41.4 107.44,41.4 IC5.30 | IC1.16 114.05,30.73 v110.49,30.73
DB5  (via drill 0.25)
  Top 0.305: v110.49,25.91 109.22,27.18 109.22,33.02 | 109.22,33.02 109.22,38.1 IC5.29 | v55.88,25.4 59.69,29.21 59.69,36.32 v65.28,41.91 | v105.41,33.02 109.22,33.02 | v77.98,33.02 76.71,34.29 v76.71,39.12
  Bottom 0.305: IC1.17 116.33,25.91 v110.49,25.91 | IC2.14 48.26,25.4 v55.88,25.4 | v65.28,41.91 IC3.15 71.63,41.4 74.42,41.4 v76.71,39.12 | v77.98,33.02 v105.41,33.02
DB6  (via drill 0.25)
  Top 0.305: IC1.18 115.57,24.13 115.57,30.73 v112.27,34.04 | v55.88,17.78 60.45,22.35 60.45,35.81 v61.47,36.83 | IC5.28 95,23.88 v95,19.3
  Bottom 0.305: v112.27,34.04 109.47,36.83 IC5.28 | IC2.17 48.26,17.78 v55.88,17.78 57.15,17.78 58.17,16.76 92.46,16.76 v95,19.3 | v61.47,36.83 64.01,39.37 IC3.16
DB7  (via drill 0.25)
  Top 0.305: IC1.19 114.81,18.29 | 114.81,18.29 v112.27,15.75 | v112.27,32.77 114.81,30.23 114.81,18.29 | v66.04,36.07 63.25,33.27 v63.25,12.7
  Bottom 0.305: IC2.18 48.26,12.7 v63.25,12.7 73.91,12.7 74.42,13.21 100.08,13.21 102.62,15.75 v112.27,15.75 | IC5.27 109.47,32.77 v112.27,32.77 | IC3.17 70.36,36.07 v66.04,36.07
E0IE10
  Top 0.305: IC8.7 82.55,62.23 82.55,71.12 IC2_DOP.7
  Bottom 0.305: IC7.15 21.59,59.69 50.8,59.69 | IC9.7 50.8,59.69 | IC8.7 82.55,59.69 50.8,59.69
GND  (via drill 0.25)
  Top 0.305: 64.77,89.41 X3.2@1 49.78,93.22 33.27,93.22 | X3.2@2 64.77,89.41 | 64.77,89.41 X3.2 83.57,83.82 83.57,82.04 85.09,80.52 85.09,71.12 | C11.2 C10.2 | C12.- 127.76,84.33 127.76,91.95 X1.2 | C9.2 99.06,73.66 X2.2 | IC3.12 IC8.8 85.09,62.23 85.09,71.12 | IC5.7 IC5.6 | 85.09,71.12 IC2_DOP.8 | IC10.7 3.81,44.45 3.81,36.83 C4.2 | 29.46,45.47 C3.2 | 29.46,45.47 29.46,54.86 C2.2 29.46,56.9 29.46,68.33 | 29.46,68.33 C1.2 31.75,68.58 R2.1 33.27,73.91 33.27,93.22 | 29.46,68.33 C14.2 | 33.27,93.22 33.27,96.27 32,97.54 S1.2 | IC4.7 29.46,28.19 29.46,45.47 | C8.2 C7.2 105.92,6.35 106.68,7.11 106.68,7.62 IC1.20 | IC12.8 55.88,50.8 55.88,59.69 IC9.8 | v54.61,5.08 IC2.1 53.34,10.16 53.34,30.48 IC2.10 IC11.8 C6.2 60.96,46.23 v57.91,49.28
  Bottom 0.305: C11.2 116.84,83.82 C12.- | C9.2 IC2_DOP.8 | IC3.12 91.44,52.07 IC5.7 | IC5.6 IC5.35 | C10.2 114.05,78.49 105.16,78.49 104.65,78.99 102.62,78.99 101.09,77.47 X2.2 | IC10.6 IC10.7 | 11.43,29.21 12.7,27.94 IC6.7 | 11.43,29.21 C4.2 | 11.43,29.21 27.94,29.21 IC4.7 35.81,34.54 51.56,34.54 54.36,31.75 IC2.10 | T2.E 9.91,97.54 16.51,97.54 S2.2 16.76,97.54 18.03,96.27 30.48,96.27 31.75,97.54 S1.2 | C3.2 38.1,44.45 IC11.15 | C2.2 38.1,55.88 IC12.15 | IC7.8 6.35,69.85 16.51,69.85 | IC7.3 16.51,69.85 | R2.1 R8.1 | 16.51,69.85 16.51,74.93 C14.2 | IC9.4 45.72,62.23 53.34,62.23 IC9.8 | C5.2 v54.61,5.08 55.37,4.32 99.06,4.32 99.31,4.57 101.09,4.57 C7.2 | IC3.18 72.39,35.56 72.39,38.1 64.01,38.1 61.72,35.81 56.9,35.81 IC11.8 | IC12.8 54.86,49.28 v57.91,49.28
IN0  (via drill 0.25)
  Top 0.305: IC1.27 127,38.1 v127,77.47 127,90.93 125.73,92.2 125.73,93.98 X1.3
  Bottom 0.305: v127,77.47 X2.3
IN1  (via drill 0.25)
  Top 0.305: IC1.28 129.54,38.1 129.54,94.49 127.51,96.52 123.19,96.52 123.19,93.98 X1.6 v118.11,88.9
  Bottom 0.305: X2.6 100.33,88.9 v118.11,88.9
IN2  (via drill 0.25)
  Top 0.305: v109.73,58.42 109.73,76.96 X2.7 106.68,93.98 118.11,93.98 X1.7
  Bottom 0.305: IC1.29 118.11,52.07 116.08,52.07 v109.73,58.42
IN3  (via drill 0.25)
  Top 0.305: IC1.30 133.35,39.37 133.35,32.51 132.59,31.75 131.57,31.75 124.46,38.86 v124.46,81.53 X1.4
  Bottom 0.305: X2.4 98.04,81.53 v124.46,81.53
IN4
  Top 0.305: X2.5 105.92,84.33 105.92,96.77 106.68,97.54 121.92,97.54 X1.5
  Bottom 0.305: IC1.31 135.13,46.23 135.13,96.52 123.19,96.52 X1.5
MA0
  Bottom 0.305: IC13.5 17.78,46.99 18.54,46.99 19.05,46.48 19.05,41.91 53.09,41.91 53.34,42.16 53.85,42.16 54.61,41.4 54.61,40.13 46.48,40.13 IC11.4
MA1  (via drill 0.25)
  Top 0.305: v50.55,42.93 52.07,41.4 IC11.7
  Bottom 0.305: IC13.7 20.32,46.99 22.35,46.99 26.42,42.93 v50.55,42.93
MA2  (via drill 0.25)
  Top 0.305: v53.59,41.15 54.61,42.16 IC11.9
  Bottom 0.305: IC13.6 16.51,50.8 14.48,50.8 13.97,50.29 13.97,41.15 v53.59,41.15
MA3  (via drill 0.25)
  Top 0.305: IC13.12 21.59,50.8 21.59,49.02 v23.11,47.5
  Bottom 0.305: v23.11,47.5 23.62,46.99 45.72,46.99 IC11.12
MA4  (via drill 0.25)
  Top 0.305: v23.62,51.31 IC13.11
  Bottom 0.305: v23.62,51.31 26.67,48.26 43.18,48.26 IC12.4
MA5  (via drill 0.25)
  Top 0.305: IC13.10 23.62,53.85 v23.62,52.83
  Bottom 0.305: v23.62,52.83 24.38,52.07 49.53,52.07 IC12.7
MA6
  Bottom 0.305: IC13.13 15.24,54.61 42.67,54.61 43.18,54.1 51.31,54.1 54.36,57.15 IC12.9
MA7
  Bottom 0.305: IC13.9 34.8,57.15 36.07,58.42 45.72,58.42 IC12.12
MA8
  Bottom 0.305: IC13.1 5.08,55.88 4.32,55.88 3.81,56.39 3.81,76.2 36.07,76.2 37.85,77.98 71.63,77.98 IC2_DOP.14
N$1
  Bottom 0.305: IC9.10 53.34,69.85 65.53,69.85 66.04,69.34 67.31,69.34 67.82,69.85 69.85,69.85 IC8.15
N$2
  Top 0: 0,0.25 0,-0.25
N$3
  Top 0: -0.25,0.1 -0.1,0.25 0.1,0.25 0.25,0.1 0.25,-0.1 0.1,-0.25 -0.1,-0.25 -0.25,-0.1 -0.25,0.1
N$4
  Bottom 0.305: C13.2 C15.2
N$5
  Top 0: 128.27,85.34 128.27,79.76
N$7
  Top 0: 46.99,87.63 46.99,90.02 46.99,92.86 46.99,95.25
N$8
  Top 0: 34.29,95 34.29,87.88
N$9
  Top 0: 19.05,95 19.05,87.88
N$14
  Top 0.305: IC10.1 19.05,46.99 19.05,51.56 13.97,56.64 13.97,59.69 IC7.12
N$15  (via drill 0.25)
  Top 0.305: IC4.1 IC4.2 | Q2.1 121.67,74.68 121.67,80.52 v112.27,89.92
  Bottom 0.305: 11.43,11.43 R3.1 | 11.43,11.43 27.94,11.43 IC4.1 | v112.27,89.92 112.01,90.17 68.83,90.17 64.01,95 9.4,95 7.11,92.71 5.59,92.71 2.29,89.41 2.29,11.43 11.43,11.43
N$16
  Top 0.305: 21.34,11.18 21.59,11.43 27.94,11.43 27.94,16.51 IC4.3 | 21.34,11.18 R3.2 | R6.1 16.26,33.27 16.26,16.26 21.34,11.18
  Bottom 0.305: IC4.5 IC4.4 IC4.3
N$17  (via drill 0.25)
  Top 0.305: v108.71,74.93 98.55,64.77 v98.55,53.59 | IC4.6 25.4,29.21 R6.2
  Bottom 0.305: IC4.10 IC4.9 IC4.6 | IC10.9 8.89,39.37 11.43,39.37 | 11.43,39.37 13.46,39.37 13.97,38.86 13.97,36.32 11.68,36.32 10.16,34.8 10.16,31.24 19.05,31.24 20.07,30.23 21.34,30.23 R6.2 | Q2.2 124.46,74.93 v108.71,74.93 | v98.55,53.59 98.3,53.34 53.09,53.34 52.83,53.09 24.64,53.09 23.88,53.85 14.99,53.85 11.43,50.29 11.43,39.37
N$38  (via drill 0.25)
  Top 0.305: v17.78,8.89 IC6.1 | v88.65,9.14 93.98,14.48 93.98,33.02 IC5.14
  Bottom 0.305: v17.78,8.89 18.8,7.87 45.97,7.87 46.23,7.62 87.12,7.62 v88.65,9.14
N$39  (via drill 0.25)
  Top 0.305: IC4.12 20.32,19.05 v20.32,31.24 | v89.15,36.58 91.44,34.29 91.44,33.02 IC5.15
  Bottom 0.305: v20.32,31.24 25.91,36.83 37.59,36.83 38.1,37.34 38.1,39.37 42.67,39.37 43.18,38.86 43.18,36.83 47.75,36.83 48.26,37.34 48.26,39.37 59.18,39.37 60.45,40.64 73.91,40.64 76.45,38.1 87.12,38.1 88.65,36.58 v89.15,36.58
N$66  (via drill 0.25)
  Top 0.305: v75.95,65.28 76.2,65.53 76.2,66.04 76.96,66.8 78.23,66.8 78.23,62.23 77.47,61.47 77.47,59.18 75.95,57.66 75.95,57.15 76.71,56.39 85.34,56.39 v85.34,59.44
  Bottom 0.305: IC13.14 10.16,59.69 9.4,59.69 8.89,60.2 8.89,64.01 41.66,64.01 42.93,65.28 v75.95,65.28 | v85.34,59.44 85.6,59.69 90.68,59.69 91.95,60.96 111.76,60.96 IC1.1
N$67
  Bottom 0.305: C13.1 46.99,78.74 31.75,78.74 R1.2
N$69
  Top 0.305: R7.3 45.47,91.44 45.47,91.69 44.7,92.46 35.31,92.46 35.31,82.8 R8.2
N$70
  Top 0.305: R7.1 40.64,87.63 40.64,73.66 R9.1
N$71
  Top 0.305: 26.16,76.71 27.94,74.93 R1.1 | 26.16,76.71 C14.1 | R2.2 26.16,76.96 26.16,76.71
  Bottom 0.305: T1.B 5.08,78.74 21.59,78.74 C14.1
N$72
  Top 0.305: C10.1 118.11,77.47 118.11,64.77 IC1.2
  Bottom 0.305: Q1.1 26.16,0.51 116.84,0.51 133.35,17.02 133.35,41.91 130.3,41.91 117.6,54.61 116.08,54.61 115.57,55.12 115.57,63.5 IC1.2
N$73  (via drill 0.25)
  Top 0.305: IC4.13 27.94,21.59 32.26,21.59 32.26,63.75 v35.56,67.06 | IC1.39 133.35,64.77 v133.35,68.07
  Bottom 0.305: v35.56,67.06 35.81,67.31 38.1,67.31 | 38.1,67.31 43.18,67.31 IC9.13 | v133.35,68.07 125.48,75.95 90.68,75.95 89.92,75.18 50.29,75.18 48.26,73.15 42.16,73.15 38.86,69.85 38.61,69.85 38.1,69.34 38.1,67.31
N$74  (via drill 0.25)
  Top 0.305: C11.1 122.43,83.31 122.43,66.55 IC1.3 111.25,55.37 111.25,32.51 111.51,32.26 111.51,16.26 v109.98,14.73
  Bottom 0.305: Q1.2 28.7,7.11 45.97,7.11 46.23,6.86 96.52,6.86 104.39,14.73 v109.98,14.73
N$75  (via drill 0.25)
  Top 0.305: C12.+ 128.02,81.03 v128.02,69.09
  Bottom 0.305: v128.02,69.09 117.35,58.42 IC1.4
N$76
  Bottom 0.305: IC5.5 92.96,56.9 106.17,56.9 107.19,55.88 108.71,55.88 116.33,48.26 IC1.8
N$77  (via drill 0.25)
  Top 0.305: v74.68,32.77 IC3.20 | v105.66,39.12 v102.11,35.56
  Bottom 0.305: v74.68,32.77 77.47,35.56 v102.11,35.56 | v105.66,39.12 107.19,40.64 111.76,40.64 IC1.9
N$78  (via drill 0.25)
  Top 0.305: IC1.10 115.06,44.96 v115.06,50.8
  Bottom 0.305: v115.06,50.8 108.71,57.15 IC5.36
N$79  (via drill 0.25)
  Top 0.305: v118.11,24.13 118.11,39.37 IC1.11
  Bottom 0.305: IC2.11 45.72,30.48 45.72,27.94 89.41,27.94 91.95,25.4 109.73,25.4 111,24.13 v118.11,24.13
N$85  (via drill 0.25)
  Top 0.305: IC6.2 15.24,16.51 15.24,32.51 13.97,33.78 13.97,40.13 8.89,45.21 8.89,62.99 11.43,65.53 | 11.43,65.53 13.97,68.07 13.97,71.12 R5.1 | IC1.34 130.3,52.58 130.3,94.49 126.49,98.3 50.29,98.3 v50.29,93.98 | 11.43,65.53 8.89,68.07 8.89,88.9 T2.C
  Bottom 0.305: v50.29,93.98 49.02,92.71 12.19,92.71 10.92,91.44 T2.C
N$86
  Top 0.305: R4.1 13.97,77.47 13.97,89.41 14.22,89.66 14.22,90.17 11.68,92.71 5.08,92.71 5.08,90.17 T2.B
N$87
  Bottom 0.305: T1.C 7.62,81.28 17.78,81.28 R4.2
PEIE10
  Top 0.305: IC2_DOP.9 87.63,78.74 87.63,69.85 IC8.9 | IC6.3 12.45,19.3 12.45,36.58 11.43,37.59 11.43,40.13 6.35,45.21 6.35,50.04 3.81,52.58 3.81,59.69 IC7.9
  Bottom 0.305: IC8.9 85.09,67.31 55.88,67.31 IC9.9 52.07,66.04 10.16,66.04 IC7.9
RAS
  Top 0.305: IC10.13 13.97,41.91 13.97,48.26 IC13.4
S
  Top 0.305: IC12.1 35.56,48.26 35.56,39.37 IC11.1
  Bottom 0.305: IC10.12 16.51,39.37 28.7,39.37 29.97,38.1 IC11.1
SA0  (via drill 0.25)
  Top 0.305: v33.27,58.17 34.8,56.64 34.8,38.1 40.39,32.51 41.91,32.51 IC11.3
  Bottom 0.305: IC7.11 12.7,58.42 33.02,58.42 v33.27,58.17
SA1  (via drill 0.25)
  Top 0.305: v69.34,35.05 69.34,57.4 72.39,60.45 72.39,67.31 IC8.14
  Bottom 0.305: IC11.6 52.58,35.05 v69.34,35.05
SA2  (via drill 0.25)
  Top 0.305: v71.88,51.05 74.93,54.1 74.93,67.31 IC8.13
  Bottom 0.305: IC11.10 54.61,48.26 69.09,48.26 v71.88,51.05
SA3  (via drill 0.25)
  Top 0.305: IC11.13 45.72,46.99 45.72,50.04 46.48,50.8 47.75,50.8 47.75,50.55 48.26,50.04 48.26,49.02 49.02,48.26 56.9,48.26 56.9,60.96 v66.29,70.36
  Bottom 0.305: v66.29,70.36 66.55,70.61 76.71,70.61 IC8.12
SA4  (via drill 0.25)
  Top 0.305: IC12.3 43.43,51.05 v43.43,55.12 | v76.96,57.4 80.01,60.45 80.01,67.31 IC8.11
  Bottom 0.305: v43.43,55.12 44.2,55.88 50.29,55.88 50.8,56.39 50.8,58.42 66.55,58.42 67.56,57.4 v76.96,57.4
SA5
  Top 0.305: IC12.6 48.51,50.55 48.51,51.31 43.18,56.64 43.18,67.31 IC9.14
SA6
  Top 0.305: IC12.10 51.56,57.66 51.56,59.69 50.8,60.45 50.8,69.09 50.04,69.85 46.99,69.85 IC9.12
SA7
  Top 0.305: IC12.13 45.72,58.42 45.72,64.77 IC9.11
VCC  (via drill 0.25)
  Top 0.305: C7.1 C8.1 97.79,21.59 IC5.26 | v131.32,91.95 132.08,91.19 IC1.40 | IC1.26 118.11,44.45 118.11,54.61 IC1.5 | IC3.24 69.85,20.32 69.85,25.4 IC3.21 68.33,29.46 68.33,42.42 68.58,42.67 68.58,46.99 | 68.58,46.99 C6.1 | 68.58,46.99 IC8.1 IC8.16 67.31,69.85 67.31,72.14 | IC2_DOP.16 67.31,78.74 67.31,72.14 | 7.62,34.29 7.37,34.29 7.37,35.81 IC10.8 | 7.62,34.29 C4.1 | C5.1 40.89,5.08 40.89,4.57 41.4,4.06 46.99,4.06 IC2.20 | 7.62,34.29 7.62,13.97 IC6.14 | IC7.10 IC7.7 7.62,73.66 T1.E | IC11.16 38.1,46.99 38.1,55.88 IC12.16 35.56,58.42 35.56,65.79 36.83,67.06 36.83,68.07 | C3.1 31.5,40.39 31.5,49.78 C2.1 31.5,51.82 31.5,61.21 C1.1 | IC7.16 IC7.1 22.86,70.36 21.84,71.37 21.84,75.95 R5.2 | R9.2 36.83,80.01 IC9.16 36.83,68.07 | 67.31,72.14 40.64,72.14 40.64,71.88 36.83,68.07 | X2.1 v93.98,71.37
  Bottom 0.305: IC1.26 130.81,31.75 IC5.26 | 93.98,69.85 85.09,69.85 IC8.10 | 93.98,69.85 100.33,69.85 C9.1 105.16,70.1 128.27,70.1 129.03,69.34 129.03,66.04 | IC1.5 127,66.04 129.03,66.04 | IC1.40 129.03,66.04 | X1.1 130.3,91.95 v131.32,91.95 | X2.1 92.96,78.49 89.92,78.49 87.12,81.28 69.85,81.28 IC2_DOP.16 | IC10.14 17.78,35.56 12.7,35.56 C4.1 | IC6.14 7.62,13.97 20.32,13.97 | IC4.14 20.32,13.97 | IC2.20 41.91,13.97 20.32,13.97 | C1.1 29.97,61.72 23.62,61.72 IC7.16 | IC9.16 IC7.1 21.59,67.31 8.89,67.31 IC7.7 | IC10.8 5.08,44.45 4.32,44.45 3.81,44.96 3.81,48.26 5.84,48.26 6.35,48.77 6.35,60.96 IC7.10 | v93.98,71.37 93.98,69.85
VCCIE10  (via drill 0.25)
  Top 0.305: IC9.1 40.64,64.77 40.64,69.09 42.67,71.12 v55.88,71.12
  Bottom 0.305: v55.88,71.12 56.39,71.63 67.82,71.63 IC2_DOP.1
VIDEO  (via drill 0.25)
  Top 0.305: R7.2 43.18,85.09 C15.1 | IC13.2 6.35,50.8 6.35,70.1 5.08,71.37 v5.08,81.28
  Bottom 0.305: v5.08,81.28 12.7,88.9 R7.2 | X3.1 62.23,81.28 44.45,81.28 C15.1
WE
  Top 0.305: IC4.11 22.86,19.05 22.86,17.27 22.1,16.51 17.02,16.51 17.02,37.08 16.51,37.59 16.51,38.61 11.43,43.69 11.43,48.26 IC13.3

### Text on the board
_tplace: 2 | 2 | 1
_tNames: X1 | X1 | X1 | R10 | R10 | R10 | X3 | X3 | X3 | T2 | T2 | T2 | S2 | S2 | S2 | S1 | S1 | S1 | C14 | C14 | C14 | C13 | C13 | C13 | R3 | R3 | R3 | R4 | R4 | R4 | C15 | C15 | C15 | R5 | R5 | R5 | R6 | R6 | R6 | R7 | R7 | R7 | R8 | R8 | R8 | C2 | C2 | C2 | C1 | C1 | C1 | T1 | T1 | T1 | C12 | C12 | C12 | X2 | X2 | X2 | IC2_DOP | IC2_DOP | IC2_DOP | Q2 | Q2 | Q2 | C11 | C11 | C11 | IC11 | IC11 | IC11 | IC13 | IC13 | IC13 | IC1 | IC1 | IC1 | IC2 | IC2 | IC2 | IC3 | IC3 | IC3 | C3 | C3 | C3 | IC12 | IC12 | IC12 | IC4 | IC4 | IC4 | C4 | C4 | C4 | IC6 | IC6 | IC6 | IC5 | IC5 | IC5 | C5 | C5 | C5 | C8 | C8 | C8 | R2 | R2 | R2 | C6 | C6 | C6 | IC10 | IC10 | IC10 | C10 | C10 | C10 | IC9 | IC9 | IC9 | IC8 | IC8 | IC8 | C9 | C9 | C9 | C7 | C7 | C7 | R1 | R1 | R1 | IC7 | IC7 | IC7 | Q1 | Q1 | Q1
DrillLegend: LAYER-STACK
DrillLegend_01-16: 01-16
